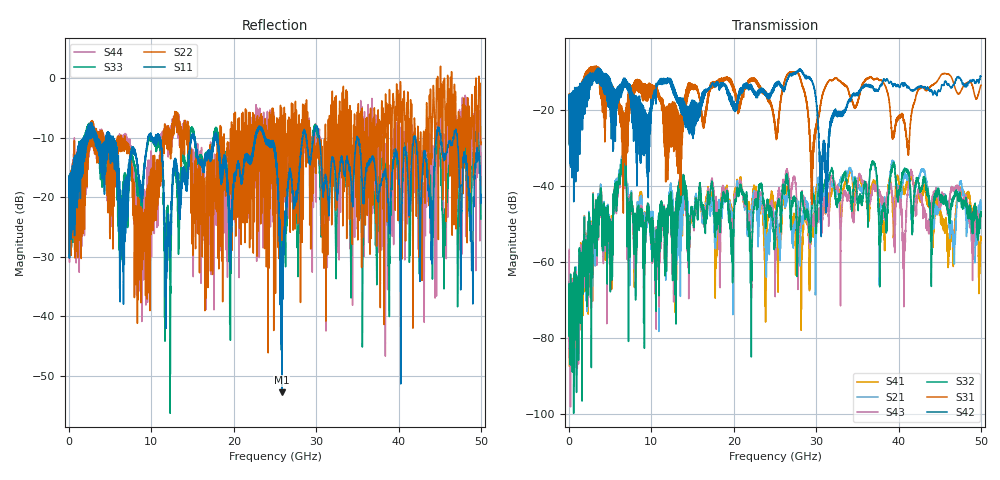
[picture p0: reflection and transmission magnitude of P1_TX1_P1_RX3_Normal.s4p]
!Keysight Technologies,N5225B,MY57041031,A.13.20.10
!Date: Friday, May 31, 2019 11:17:05
!Correction: S11(Full 4 Port(1,2,3,4))
!S12(Full 4 Port(1,2,3,4))
!S13(Full 4 Port(1,2,3,4))
!S14(Full 4 Port(1,2,3,4))
!S21(Full 4 Port(1,2,3,4))
!S22(Full 4 Port(1,2,3,4))
!S23(Full 4 Port(1,2,3,4))
!S24(Full 4 Port(1,2,3,4))
!S31(Full 4 Port(1,2,3,4))
!S32(Full 4 Port(1,2,3,4))
!S33(Full 4 Port(1,2,3,4))
!S34(Full 4 Port(1,2,3,4))
!S41(Full 4 Port(1,2,3,4))
!S42(Full 4 Port(1,2,3,4))
!S43(Full 4 Port(1,2,3,4))
!S44(Full 4 Port(1,2,3,4))
!S4P File: Measurements: <S11,S12,S13,S14>,
!<S21,S22,S23,S24>,
!<S31,S32,S33,S34>,
!<S41,S42,S43,S44>:
# Hz S  dB  R 50.0
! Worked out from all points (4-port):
!   5000 points, 10 MHz to 50 GHz, reference 50 ohm
!   strongest paths, dB at 10 MHz, 12.51 GHz, 25.01 GHz, 37.51 GHz, 50 GHz:
!     S42: -19.6, -14.4, -13.4, -15.0, -11.2
!     S31: -19.4, -29.3, -24.6, -11.8, -13.5
!     S32: -79.4, -47.0, -54.2, -42.8, -47.3
!     S43: -56.7, -48.6, -59.3, -41.6, -47.1
!     S21: -57.2, -43.2, -47.9, -43.7, -45.4
!     S41: -62.9, -44.8, -44.4, -43.0, -53.7
!   lowest |S11| = -52.7 dB at 25.83 GHz (marker M1), VSWR 1.00, Z = 50 + j0.23 ohm
!   |S11| at or under -10 dB: 18.01 GHz to 22.61 GHz (4.596 GHz wide, 22.6 % of centre); 30.38 GHz to 34.94 GHz (4.563 GHz wide, 14 % of centre); 34.98 GHz to 41.82 GHz (6.842 GHz wide, 17.8 % of centre)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
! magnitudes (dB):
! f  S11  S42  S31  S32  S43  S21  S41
! 10 MHz  -19.9  -19.6  -19.4  -79.4  -56.7  -57.2  -62.9
! 6.49 GHz  -21.1  -13.1  -32.5  -33.0  -33.6  -32.3  -32.6
! 10.44 GHz  -10.5  -15.9  -15.5  -57.6  -56.5  -54.2  -55.1
! 23.21 GHz  -8.2  -15.3  -14.3  -40.0  -42.6  -43.4  -44.8
! 25.83 GHz  -52.7  -14.3  -16.0  -43.5  -43.0  -44.9  -50.0
! 30.63 GHz  -14.3  -40.6  -17.6  -40.7  -51.4  -42.8  -44.0
! 50 GHz  -19.5  -11.2  -13.5  -47.3  -47.1  -45.4  -53.7
